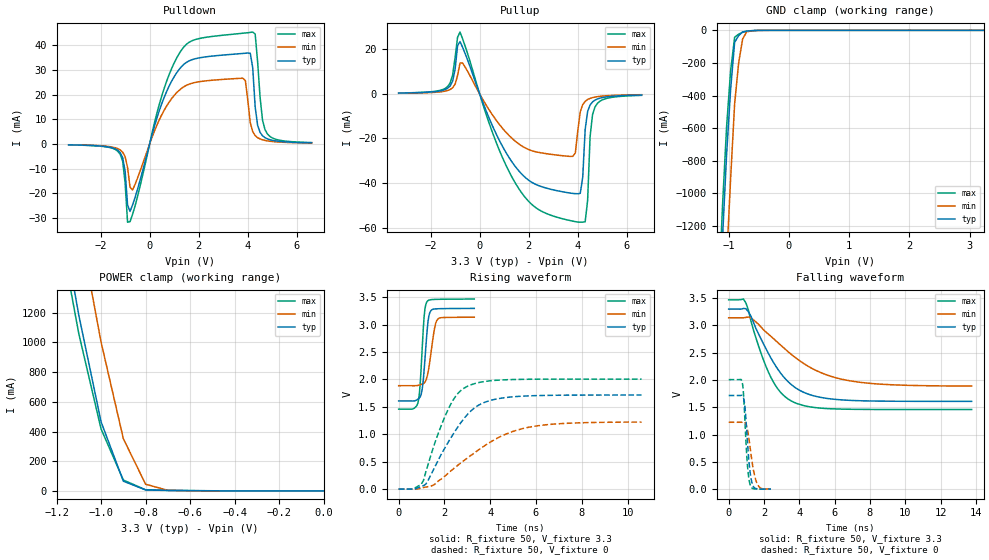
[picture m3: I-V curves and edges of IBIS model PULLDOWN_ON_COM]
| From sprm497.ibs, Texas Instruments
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|   Model Cell PULLDOWN_ON_COM
[Model]   PULLDOWN_ON_COM
Model_type   I/O
Polarity   Non-Inverting
Enable   Active-Low
Vinl =  0.8
Vinh =  2
Cref =  15.0000pF
Rref =  100.0000M
Vref =  0V
Vmeas =  1.65
C_comp   0.8695239p   0.8563616p   0.8781626p
[Model Spec]
Vinl   0.8   0.8   0.8
Vinh   2   2   2
[Temperature Range]   25   105   0
[Voltage Range]   3.3   3.14   3.47
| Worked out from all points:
|   slope of the pulldown table from 0 to 0.495 V, typ, clamps not added: 30.2 ohm
|   slope of the pullup table from 0 to 0.495 V, typ, clamps not added: 36.2 ohm
|   GND clamp passes 1 mA (typ) near -0.57 V on its own axis
|   POWER clamp passes 1 mA (typ) near -0.51 V on its own axis
|   rising waveform, R_fixture 50, V_fixture 3.3: 20-80 % time 196ps typ, 262ps min, 170ps max; typ from 1.61 V to 3.3 V
|   rising waveform, R_fixture 50, V_fixture 0: 20-80 % time 1.52ns typ, 2.51ns min, 1.1ns max; typ from 0 V to 1.72 V
|   falling waveform, R_fixture 50, V_fixture 3.3: 20-80 % time 1.92ns typ, 3.11ns min, 1.46ns max; typ from 3.3 V to 1.61 V
|   falling waveform, R_fixture 50, V_fixture 0: 20-80 % time 245ps typ, 349ps min, 206ps max; typ from 1.72 V to 0.002 V
[POWER_clamp]
|   voltage   I(typ)   I(min)   I(max)
-3.3V     22.37A     22.96A     22.21A
-1.133V   1.464A     2.096A     1.329A
-1.1V     1.183A     1.806A     1.058A
-1.067V   943.8mA    1.538A     844.6mA
-1.033V   704.5mA    1.27A      631mA
-1V       465.3mA    1.002A     417.3mA
-900mV    65.82mA    351.8mA    73.35mA
-800mV    6.559mA    45.11mA    7.857mA
-700mV    3.243mA    4.096mA    4.125mA
-11.55fV  93.69uA    61.44uA    121.1uA
[Pulldown]
|   voltage   I(typ)   I(min)   I(max)
-3.3V     -379.4uA   -345.5uA   -405uA
-1.3V     -2.568mA   -1.909mA   -2.955mA
-1.1V     -5.533mA   -3.354mA   -7.005mA
-900mV    -24.8mA    -9.58mA    -31.78mA
-800mV    -27.41mA   -17.54mA   -31.56mA
400mV     13.7mA     9.942mA    16.3mA
1.2V      30.21mA    21.74mA    36.6mA
3.8V      36.73mA    26.64mA    44.94mA
4.2V      30.93mA    4.999mA    45.4mA
4.4V      7.557mA    2.538mA    33.36mA
4.7V      2.533mA    1.415mA    5.821mA
6.6V      436uA      357.4uA    548uA
[Pullup]
|   voltage   I(typ)   I(min)   I(max)
-3.3V     352.6uA    268.9uA    395.9uA
-1.3V     2.559mA    1.54mA     3.337mA
-800mV    23.47mA    13.87mA    27.72mA
1.5V      -33.25mA   -21.66mA   -40.85mA
3.8V      -44.66mA   -28.01mA   -57.09mA
4.1V      -44.61mA   -8.068mA   -57.55mA
4.2V      -37.49mA   -4.806mA   -57.56mA
4.3V      -15.99mA   -3.326mA   -57.36mA
4.4V      -7.897mA   -2.517mA   -47.82mA
4.5V      -4.997mA   -2.014mA   -19.22mA
4.7V      -2.803mA   -1.431mA   -5.878mA
6.6V      -515.4uA   -371.2uA   -665.4uA
[GND_clamp]
|   voltage   I(typ)   I(min)   I(max)
-3.3V     -22.52A    -23.16A    -22.34A
-1.167V   -1.845A    -2.552A    -1.643A
-1.1V     -1.269A    -1.966A    -1.072A
-1.033V   -763.9mA   -1.418A    -593.7mA
-966.7mV  -365.3mA   -913.8mA   -250.4mA
-900mV    -73.59mA   -452.5mA   -42.5mA
-833.3mV  -32.67mA   -200.8mA   -23.36mA
-766.7mV  -9.715mA   -52.91mA   -11.18mA
-700mV    -4.738mA   -8.897mA   -5.952mA
-500mV    -215.1uA   -459uA     -253.2uA
3.233V    93.67uA    61.57uA    121uA
[Ramp]
| variable   typ   min   max
dV/dt_f   1.023768/1.927095n   0.7595791/3.147426n   1.215988/1.459756n
dV/dt_r   1.030119/1.522204n   0.7360508/2.521247n   1.204341/1.10109n
R_load = 50
[Rising Waveform]
R_fixture = 50
V_fixture = 3.3
V_fixture_min = 3.14
V_fixture_max = 3.47
|   time   V(typ)   V(min)   V(max)
0s        1.609V     1.887V     1.46V
844ps     1.643V     1.892V     1.577V
944ps     1.686V     1.904V     1.947V
1.044ns   1.872V     1.918V     2.689V
1.148ns   2.37V      1.951V     3.285V
1.248ns   2.914V     2.062V     3.425V
1.384ns   3.239V     2.399V     3.454V
1.552ns   3.285V     2.895V     3.46V
1.688ns   3.289V     3.089V     3.462V
3.304ns   3.296V     3.135V     3.467V
[Rising Waveform]
R_fixture = 50
V_fixture = 0
V_fixture_min = 0
V_fixture_max = 0
|   time   V(typ)   V(min)   V(max)
0s        97.34nV    174.3nV    117nV
972ps     47.67mV    17.83mV    81.46mV
1.188ns   90.67mV    38.33mV    317.3mV
1.62ns    437.1mV    103.5mV    890.9mV
2.164ns   854.7mV    290.1mV    1.456V
2.596ns   1.141V     439.3mV    1.749V
3.032ns   1.374V     576.4mV    1.881V
3.896ns   1.604V     829.6mV    1.971V
5.632ns   1.7V       1.124V     2.004V
10.62ns   1.716V     1.223V     2.007V
[Falling Waveform]
R_fixture = 50
V_fixture = 3.3
V_fixture_min = 3.14
V_fixture_max = 3.47
|   time   V(typ)   V(min)   V(max)
0s        3.298V     3.138V     3.468V
840ps     3.31V      3.138V     3.482V
1.26ns    3.168V     3.136V     3.08V
1.82ns    2.76V      2.975V     2.501V
2.384ns   2.407V     2.801V     2.053V
2.944ns   2.124V     2.638V     1.772V
3.648ns   1.889V     2.442V     1.599V
5.192ns   1.683V     2.139V     1.486V
6.876ns   1.627V     1.985V     1.464V
13.75ns   1.609V     1.89V      1.46V
[Falling Waveform]
R_fixture = 50
V_fixture = 0
V_fixture_min = 0
V_fixture_max = 0
|   time   V(typ)   V(min)   V(max)
0s        1.716V     1.226V     2.007V
776ps     1.717V     1.228V     1.942V
848ps     1.665V     1.234V     1.706V
924ps     1.498V     1.222V     1.228V
1.068ns   845.8mV    1.083V     417.8mV
1.144ns   528.8mV    930.7mV    191.8mV
1.24ns    249.6mV    699.2mV    59.86mV
1.388ns   58.11mV    375.7mV    11.25mV
1.628ns   7.211mV    92.83mV    3.655mV
2.384ns   1.923mV    3.171mV    1.475mV
